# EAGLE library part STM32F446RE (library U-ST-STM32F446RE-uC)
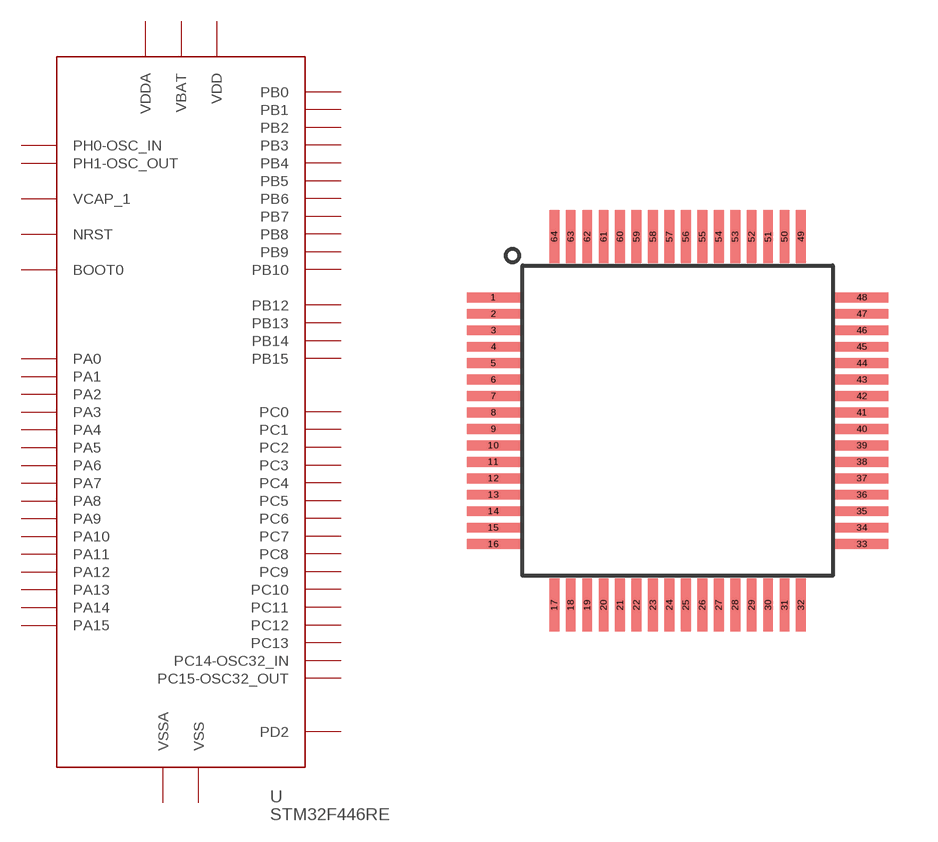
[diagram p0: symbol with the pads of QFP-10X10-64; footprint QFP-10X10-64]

Designator prefix -

## STM32F446RE  [QFP-10X10-64]
1  VBAT  pwr
2  PC13
3  PC14-OSC32_IN
4  PC15-OSC32_OUT
5  PH0-OSC_IN
6  PH1-OSC_OUT
7  NRST
8  PC0
9  PC1
10  PC2
11  PC3
12  VSSA  pwr
13  VDDA  pwr
14  PA0
15  PA1
16  PA2
17  PA3
18  VSS  pwr
19  VDD  pwr
20  PA4
21  PA5
22  PA6
23  PA7
24  PC4
25  PC5
26  PB0
27  PB1
28  PB2
29  PB10
30  VCAP_1
31  VSS  pwr
32  VDD  pwr
33  PB12
34  PB13
35  PB14
36  PB15
37  PC6
38  PC7
39  PC8
40  PC9
41  PA8
42  PA9
43  PA10
44  PA11
45  PA12
46  PA13
47  VSS  pwr
48  VDD  pwr
49  PA14
50  PA15
51  PC10
52  PC11
53  PC12
54  PD2
55  PB3
56  PB4
57  PB5
58  PB6
59  PB7
60  BOOT0
61  PB8
62  PB9
63  VSS  pwr
64  VDD  pwr

## Footprint QFP-10X10-64 (pad centres in mm)
QFP64 shrink quad flat pack, square
smd 1.6 x 0.3: 1 -5.6,3.75; 2 -5.6,3.25; 3 -5.6,2.75; 4 -5.6,2.25; 5 -5.6,1.75; 6 -5.6,1.25; 7 -5.6,0.75; 8 -5.6,0.25; 9 -5.6,-0.25; 10 -5.6,-0.75; 11 -5.6,-1.25; 12 -5.6,-1.75; 13 -5.6,-2.25; 14 -5.6,-2.75; 15 -5.6,-3.25; 16 -5.6,-3.75; 33 5.6,-3.75; 34 5.6,-3.25; 35 5.6,-2.75; 36 5.6,-2.25; 37 5.6,-1.75; 38 5.6,-1.25; 39 5.6,-0.75; 40 5.6,-0.25; 41 5.6,0.25; 42 5.6,0.75; 43 5.6,1.25; 44 5.6,1.75; 45 5.6,2.25; 46 5.6,2.75; 47 5.6,3.25; 48 5.6,3.75
smd 0.3 x 1.6: 17 -3.75,-5.6; 18 -3.25,-5.6; 19 -2.75,-5.6; 20 -2.25,-5.6; 21 -1.75,-5.6; 22 -1.25,-5.6; 23 -0.75,-5.6; 24 -0.25,-5.6; 25 0.25,-5.6; 26 0.75,-5.6; 27 1.25,-5.6; 28 1.75,-5.6; 29 2.25,-5.6; 30 2.75,-5.6; 31 3.25,-5.6; 32 3.75,-5.6; 49 3.75,5.6; 50 3.25,5.6; 51 2.75,5.6; 52 2.25,5.6; 53 1.75,5.6; 54 1.25,5.6; 55 0.75,5.6; 56 0.25,5.6; 57 -0.25,5.6; 58 -0.75,5.6; 59 -1.25,5.6; 60 -1.75,5.6; 61 -2.25,5.6; 62 -2.75,5.6; 63 -3.25,5.6; 64 -3.75,5.6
